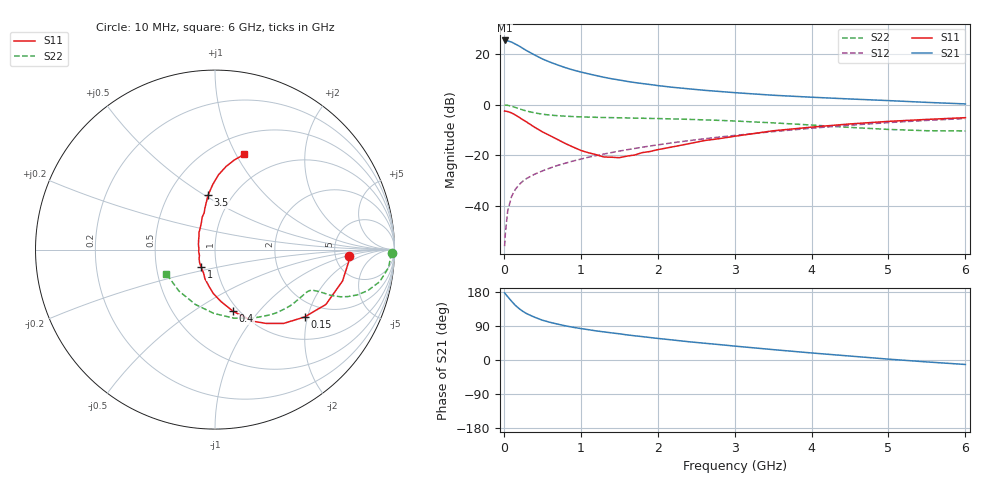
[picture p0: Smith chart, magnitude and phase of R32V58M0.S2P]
! SIEMENS Small Signal Semiconductors
! BFR181
! Si NPN RF Bipolar Junction Transistor in SOT23
! VCE = 2.5 V  IC = 8 mA
! Common Emitter S-Parameters:  May  1996
# GHz  S  MA  R  50
!  f  S11  S21  S12  S22
! GHz  MAG  ANG  MAG  ANG  MAG  ANG  MAG  ANG
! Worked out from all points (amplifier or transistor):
!   36 points, 10 MHz to 6 GHz, reference 50 ohm
!   highest |S21| = 25.4 dB at 10 MHz (marker M1)
!   |S21| within 3 dB of that: start of sweep to 240.7 MHz
!   unconditionally stable (mu >= 1): 835.8 MHz to 2.747 GHz
!   at 250 MHz: K = 0.56, MSG = 26.2 dB, |S12| = -30.1 dB
!   at 1.4 GHz: K = 1.07, MAG = 13.0 dB, |S12| = -18.9 dB
!   at 6 GHz: K = 0.85, MSG = 2.9 dB, |S12| = -5.5 dB
!   S11 on the Smith chart (normalised r, x): 10 MHz: 6.79, -1.18; 150 MHz: 1.55, -1.91; 400 MHz: 0.94, -0.74; 1 GHz: 0.84, -0.17; 3.5 GHz: 0.77, +0.52; 6 GHz: 0.70, +1.08
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0.01  0.7499 -2.9  18.6 177.2  0.0016 92.2  0.9856 -1.1
0.02  0.747 -5.5  18.34 174.5  0.0029 84.5  0.9797 -2.3
0.05  0.7319 -13.8  18.27 167.1  0.0079 82.3  0.9721 -5.9
0.1  0.6894 -26.3  17.28 155.2  0.0153 77.8  0.9353 -11.0
0.15  0.6244 -37.0  15.78 144.1  0.0213 72.4  0.8819 -15.0
0.2  0.5614 -47.1  14.38 135.4  0.0264 71.0  0.8312 -17.7
0.25  0.501 -55.2  12.9 128.0  0.0311 67.7  0.7845 -19.5
0.3  0.451 -62.2  11.61 122.0  0.0351 67.2  0.7472 -20.6
0.4  0.358 -73.7  9.605 112.9  0.0423 66.3  0.6899 -21.6
0.5  0.2912 -83.4  8.037 105.1  0.0491 66.4  0.6493 -21.8
0.6  0.2447 -92.3  6.945 99.5  0.056 66.7  0.6233 -22.0
0.7  0.2045 -99.9  6.095 94.6  0.0632 67.5  0.606 -22.3
0.8  0.1708 -109.3  5.395 90.2  0.0698 67.4  0.5933 -22.5
1  0.1249 -127.8  4.429 83.0  0.084 68.4  0.5751 -23.4
1.1  0.1123 -139.6  4.074 80.0  0.0916 68.4  0.5684 -24.1
1.3  0.0926 -159.3  3.485 74.2  0.106 68.3  0.5582 -25.7
1.6  0.0963 163.3  2.893 66.3  0.1287 67.6  0.5475 -28.8
2.2  0.1473 123.8  2.203 52.7  0.1775 64.9  0.5235 -36.6
3.5  0.3049 97.3  1.538 27.4  0.2938 54.7  0.4376 -60.7
4.5  0.4165 87.4  1.297 10.4  0.3936 43.8  0.3557 -91.0
5.5  0.512 77.7  1.111 -5.1  0.4894 30.9  0.3059 -131.1
6  0.5541 73.0  1.036 -11.8  0.5325 23.7  0.3028 -153.2
